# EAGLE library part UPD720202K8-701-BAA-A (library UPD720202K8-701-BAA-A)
PD720202 is a USB host controller LSI compatible with the USB 3.0 and xHCI (eXtensible Host Controller Interface) 1.0 specifications. The system bus is compatible with the PCIe Gen2 specification. The controller provides two USB ports with LS (Low-Speed) / FS (Full-Speed) / HS (High-Speed) / SS (SuperSpeed) support.PD720202 comes in a 48-pin QFN package and has the following improvements over previous products. Reduced power consumption in low-power mode to 4.5mW, a reduction of 90% compared with Renesas Source: Datasheet
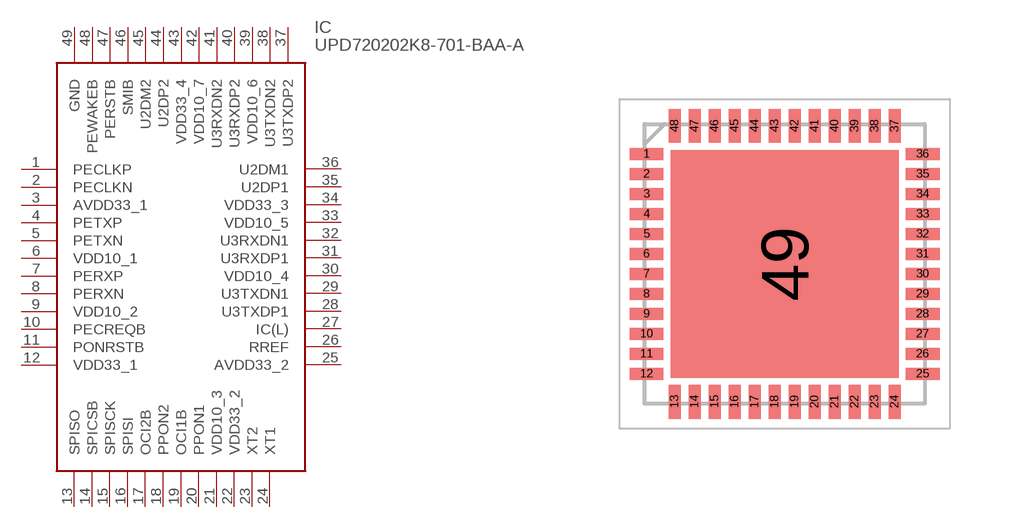
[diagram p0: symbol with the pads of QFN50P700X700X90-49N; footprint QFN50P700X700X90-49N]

Designator prefix IC

## UPD720202K8-701-BAA-A (Arrow_Part_Number: UPD720202K8-701-BAA-A; Arrow_Price-Stock: https://www.arrow.com/en/products/upd720202k8-701-baa-a/renesas-electronics; Description: PD720202 is a USB host controller LSI compatible with the USB 3.0 and xHCI (eXtensible Host Controller Interface) 1.0 specifications. The system bus is compatible with the PCIe Gen2 specification. The controller provides two USB ports with LS (Low-Speed) / FS (Full-Speed) / HS (High-Speed) / SS (SuperSpeed) support.PD720202 comes in a 48-pin QFN package and has the following improvements over previous products. Reduced power consumption in low-power mode to 4.5mW, a reduction of 90% compared with Renesas; Height: 0.9mm; Manufacturer_Name: Renesas Electronics; Manufacturer_Part_Number: UPD720202K8-701-BAA-A; Mouser_Part_Number: 968-D720202K8701BAAA; Mouser_Price-Stock: https://www.mouser.co.uk/ProductDetail/Renesas-Electronics/UPD720202K8-701-BAA-A?qs=ZVKuL1Ob8AssYP6AhEzWuA%3D%3D)  [QFN50P700X700X90-49N]
1  PECLKP
2  PECLKN
3  AVDD33_1
4  PETXP
5  PETXN
6  VDD10_1
7  PERXP
8  PERXN
9  VDD10_2
10  PECREQB
11  PONRSTB
12  VDD33_1
13  SPISO
14  SPICSB
15  SPISCK
16  SPISI
17  OCI2B
18  PPON2
19  OCI1B
20  PPON1
21  VDD10_3
22  VDD33_2
23  XT2
24  XT1
25  AVDD33_2
26  RREF
27  IC(L)
28  U3TXDP1
29  U3TXDN1
30  VDD10_4
31  U3RXDP1
32  U3RXDN1
33  VDD10_5
34  VDD33_3
35  U2DP1
36  U2DM1
37  U3TXDP2
38  U3TXDN2
39  VDD10_6
40  U3RXDP2
41  U3RXDN2
42  VDD10_7
43  VDD33_4
44  U2DP2
45  U2DM2
46  SMIB
47  PERSTB
48  PEWAKEB
49  GND

## Footprint QFN50P700X700X90-49N (pad centres in mm)
QFN-48
smd 0.85 x 0.3: 1 -3.45,2.75; 2 -3.45,2.25; 3 -3.45,1.75; 4 -3.45,1.25; 5 -3.45,0.75; 6 -3.45,0.25; 7 -3.45,-0.25; 8 -3.45,-0.75; 9 -3.45,-1.25; 10 -3.45,-1.75; 11 -3.45,-2.25; 12 -3.45,-2.75; 25 3.45,-2.75; 26 3.45,-2.25; 27 3.45,-1.75; 28 3.45,-1.25; 29 3.45,-0.75; 30 3.45,-0.25; 31 3.45,0.25; 32 3.45,0.75; 33 3.45,1.25; 34 3.45,1.75; 35 3.45,2.25; 36 3.45,2.75
smd 0.3 x 0.85: 13 -2.75,-3.45; 14 -2.25,-3.45; 15 -1.75,-3.45; 16 -1.25,-3.45; 17 -0.75,-3.45; 18 -0.25,-3.45; 19 0.25,-3.45; 20 0.75,-3.45; 21 1.25,-3.45; 22 1.75,-3.45; 23 2.25,-3.45; 24 2.75,-3.45; 37 2.75,3.45; 38 2.25,3.45; 39 1.75,3.45; 40 1.25,3.45; 41 0.75,3.45; 42 0.25,3.45; 43 -0.25,3.45; 44 -0.75,3.45; 45 -1.25,3.45; 46 -1.75,3.45; 47 -2.25,3.45; 48 -2.75,3.45
smd 5.7 x 5.7: 49 0,0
